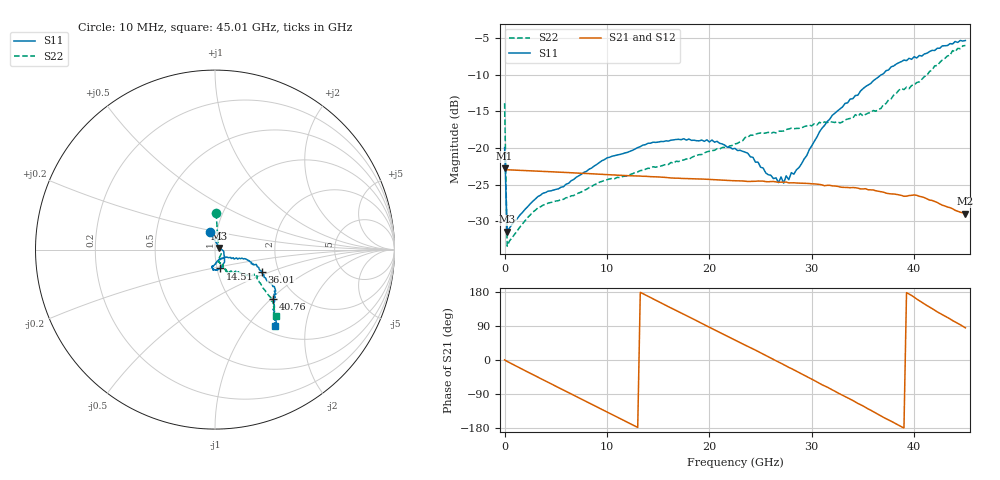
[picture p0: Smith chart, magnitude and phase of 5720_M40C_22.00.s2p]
! Device:  ADRF5720
! Description: 0.5dB LSB GaAs MMIC 6-bit Digital Attenuator
! Frequency:  0.000009 -  40 GHz
! Ports:
!	RF1	= Port 1
!	RF2	= Port 2
! Vdd:  3.3 Volt
! Vss:  -3.3 Volt
! Control:  0/3.3 Volt
! State:  22.00 dB attenuation
! Data:  The device was measured using G-S-G Probes on a matrix board.
!  Data was collected using an calibrated 4 port network analyzer.
!  The reference plane for this measurement is at the launchers.
! Note:  Analog Devices supplies this data as a sample of measured data
!  for this product.  Your particular data for this product may vary.
!  Data was taken at -40 degrees C.
!  Analog Devices reserves the right to change this data at anytime.
# GHZ S DB R 45.0
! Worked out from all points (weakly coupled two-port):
!   181 points, 10 MHz to 45.01 GHz, reference 45 ohm
!   highest |S21| = -22.80 dB at 10 MHz (marker M1); lowest = -29.0 dB at 45.01 GHz (marker M2)
!   lowest |S11| = -31.4 dB at 260 MHz (marker M3), VSWR 1.05, Z = 47.3 + j0.895 ohm
!   |S11| at or under -10 dB: start of sweep to 36.8 GHz
!   |S22| runs from -33.4 to -6.0 dB; largest |S21 - S12| = 0.00027
!   S11 on the Smith chart (normalised r, x): 10 MHz: 0.93, +0.18; 14.51 GHz: 1.04, -0.22; 36.01 GHz: 1.63, -0.44; 40.76 GHz: 1.53, -1.03; 45.01 GHz: 1.13, -1.36
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0.01  -19.95 106.8  -22.80 0.3  -22.82 0.3  -13.89 88.2
0.26  -31.45 20.7  -22.98 -3.8  -23.00 -3.8  -33.42 22.5
3.26  -26.64 -8.9  -23.17 -45.3  -23.19 -45.4  -28.19 -28.5
7.76  -23.33 -39.4  -23.47 -106.6  -23.49 -106.6  -25.80 -62.0
10.01  -21.36 -51.3  -23.64 -137.2  -23.66 -137.2  -24.33 -68.4
14.51  -19.21 -73.8  -23.93 161.4  -23.95 161.3  -22.57 -71.7
15.26  -19.12 -77.3  -23.98 151.0  -24.00 151.0  -22.48 -71.1
20.26  -18.91 -95.5  -24.32 83.0  -24.34 82.9  -20.36 -64.2
22.76  -20.35 -100.7  -24.49 49.3  -24.51 49.2  -19.37 -64.7
24.01  -21.21 -93.4  -24.57 32.7  -24.59 32.6  -18.25 -63.4
27.01  -23.96 -61.3  -24.67 -8.6  -24.70 -8.7  -17.71 -63.0
27.26  -24.81 -60.3  -24.67 -12.2  -24.69 -12.3  -17.68 -61.4
27.51  -23.81 -53.0  -24.66 -15.9  -24.67 -16.1  -17.48 -62.6
27.76  -24.34 -50.3  -24.77 -19.4  -24.79 -19.5  -17.41 -60.9
28.76  -22.67 -35.6  -24.80 -33.1  -24.82 -33.2  -17.32 -62.0
30.26  -19.08 -24.1  -24.91 -54.2  -24.94 -54.3  -16.69 -61.2
32.01  -15.54 -18.0  -25.18 -78.8  -25.21 -79.0  -16.46 -56.3
36.01  -10.82 -25.2  -25.74 -136.3  -25.77 -136.5  -14.88 -44.3
37.76  -8.91 -31.5  -26.28 -161.6  -26.30 -161.7  -13.29 -40.5
40.76  -7.44 -40.5  -26.68 152.4  -26.71 152.3  -10.60 -34.3
43.76  -5.79 -48.8  -28.31 104.0  -28.33 103.9  -6.70 -43.6
45.01  -5.32 -51.9  -28.98 84.8  -29.00 84.7  -6.00 -47.5
